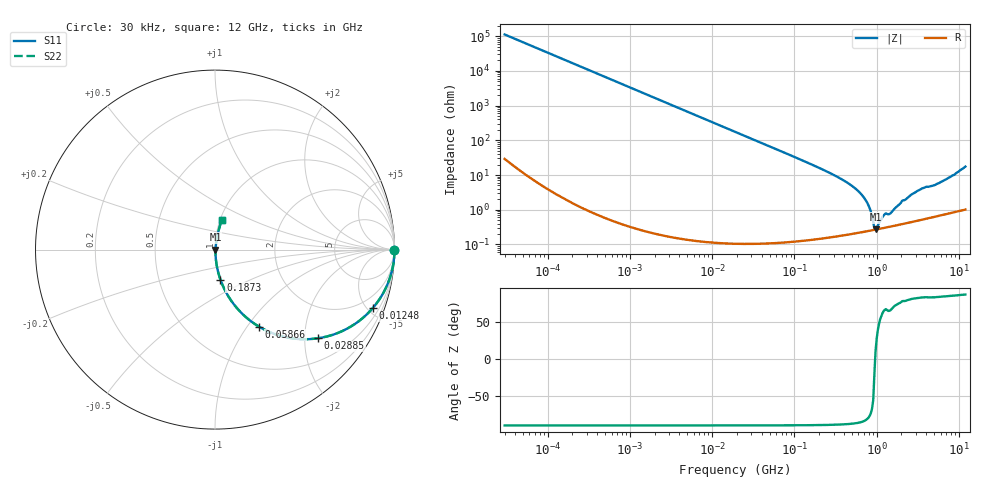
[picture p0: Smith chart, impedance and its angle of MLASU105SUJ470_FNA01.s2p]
! MLASU105SUJ470_FNA01  S-PARAMETER MODEL  ( General Type )
! Model Generated by TAIYO YUDEN Corporation (http://www.ty-top.com)
! Version 4.0
! TAIYO YUDEN Control No. 120810
! Copyright(c) 2003 TAIYO YUDEN CO.,LTD. All Rights Reserved.
! Product Description (link to TY-COMPAS)
! https://ds.yuden.co.jp/TYCOMPAS/or/detail?pn=MLASU105SUJ470JFNA01&u=M
! Products Name : Multilayer Ceramic Capacitors
! Characteristics :
!  Capacitance : 47 pF , Rated Voltage : 50V , TCC : UJ / U2J
!  Case Size : 1.0 x 0.5 / 0.039 x 0.02 [mm/inch] , Thickness : 0.5 / 0.02 [mm/inch]
!  (Conditions: Temperature = 25 degC , DC Bias Current/Voltage = 0A / 0V)
! External Node Assignments :
!  1  o---| |---o  2
! GND o---------o GND
! Frequency Range : 0.03MHz  -  12000MHz  [ 401 STEP ]
# MHz S RI R 50
! Freq[MHz].  S11 Real  S11 Imag  S21 Real  S21 Imag  S12 Real  S12 Imag  S22 Real  S22 Imag
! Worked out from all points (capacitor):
!   401 points, 30 kHz to 12 GHz, reference 50 ohm
!   read as one part in series: C = 47.3 pF near 32 kHz
!   lowest |Z| = 272 mohm at 970 MHz (marker M1)
!   series resonance near 959.9 MHz, so ESL is about 580 pH
!   S11 on the Smith chart (normalised r, x): 30 kHz: open; 12.48 MHz: 1.00, -5.39; 28.85 MHz: 1.00, -2.33; 58.66 MHz: 1.00, -1.14; 187.3 MHz: 1.00, -0.35; 12 GHz: 1.02, +0.35
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0.03  1 -0.000892  1.03e-06 0.000892  1.03e-06 0.000892  1 -0.000892
0.260295  0.9999 -0.00774  6.06e-05 0.00774  6.06e-05 0.00774  0.9999 -0.00774
2.258455  0.9955 -0.0669  0.0045 0.0669  0.0045 0.0669  0.9955 -0.0669
5.571287  0.9732 -0.1613  0.0268 0.1613  0.0268 0.1613  0.9732 -0.1613
12.47626  0.8788 -0.3262  0.1212 0.3262  0.1212 0.3262  0.8788 -0.3262
18.97367  0.7581 -0.4279  0.2419 0.4279  0.2419 0.4279  0.7581 -0.4279
28.85481  0.5752 -0.4939  0.4248 0.4939  0.4248 0.4939  0.5752 -0.4939
58.65857  0.2462 -0.4299  0.7538 0.4299  0.7538 0.4299  0.2462 -0.4299
164.6252  0.039 -0.1902  0.961 0.1902  0.961 0.1902  0.039 -0.1902
187.291  0.0302 -0.1672  0.9698 0.1672  0.9698 0.1672  0.0302 -0.1672
393.2198  0.00683 -0.0705  0.9932 0.0705  0.9932 0.0705  0.00683 -0.0705
617.6002  0.00319 -0.0317  0.9968 0.0317  0.9968 0.0317  0.00319 -0.0317
774.0045  0.00264 -0.0151  0.9974 0.0151  0.9974 0.0151  0.00264 -0.0151
825.5698  0.00259 -0.0105  0.9974 0.0105  0.9974 0.0105  0.00259 -0.0105
909.4299  0.00261 -0.00375  0.9974 0.00375  0.9974 0.00375  0.00261 -0.00375
970.0175  0.00267 0.000484  0.9973 -0.000484  0.9973 -0.000484  0.00267 0.000484
1001.808  0.00271 0.00138  0.9973 -0.00138  0.9973 -0.00138  0.00271 0.00138
1215.67  0.00301 0.00612  0.997 -0.00612  0.997 -0.00612  0.00301 0.00612
1428.372  0.00326 0.00677  0.9967 -0.00677  0.9967 -0.00677  0.00326 0.00677
2903.719  0.00553 0.0303  0.9945 -0.0303  0.9945 -0.0303  0.00553 0.0303
5534.236  0.00961 0.0553  0.9904 -0.0553  0.9904 -0.0553  0.00961 0.0553
12000  0.0388 0.1662  0.9612 -0.1662  0.9612 -0.1662  0.0388 0.1662
